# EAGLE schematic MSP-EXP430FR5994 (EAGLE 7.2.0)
DRAWN: Mike Stein; REV: 1.1

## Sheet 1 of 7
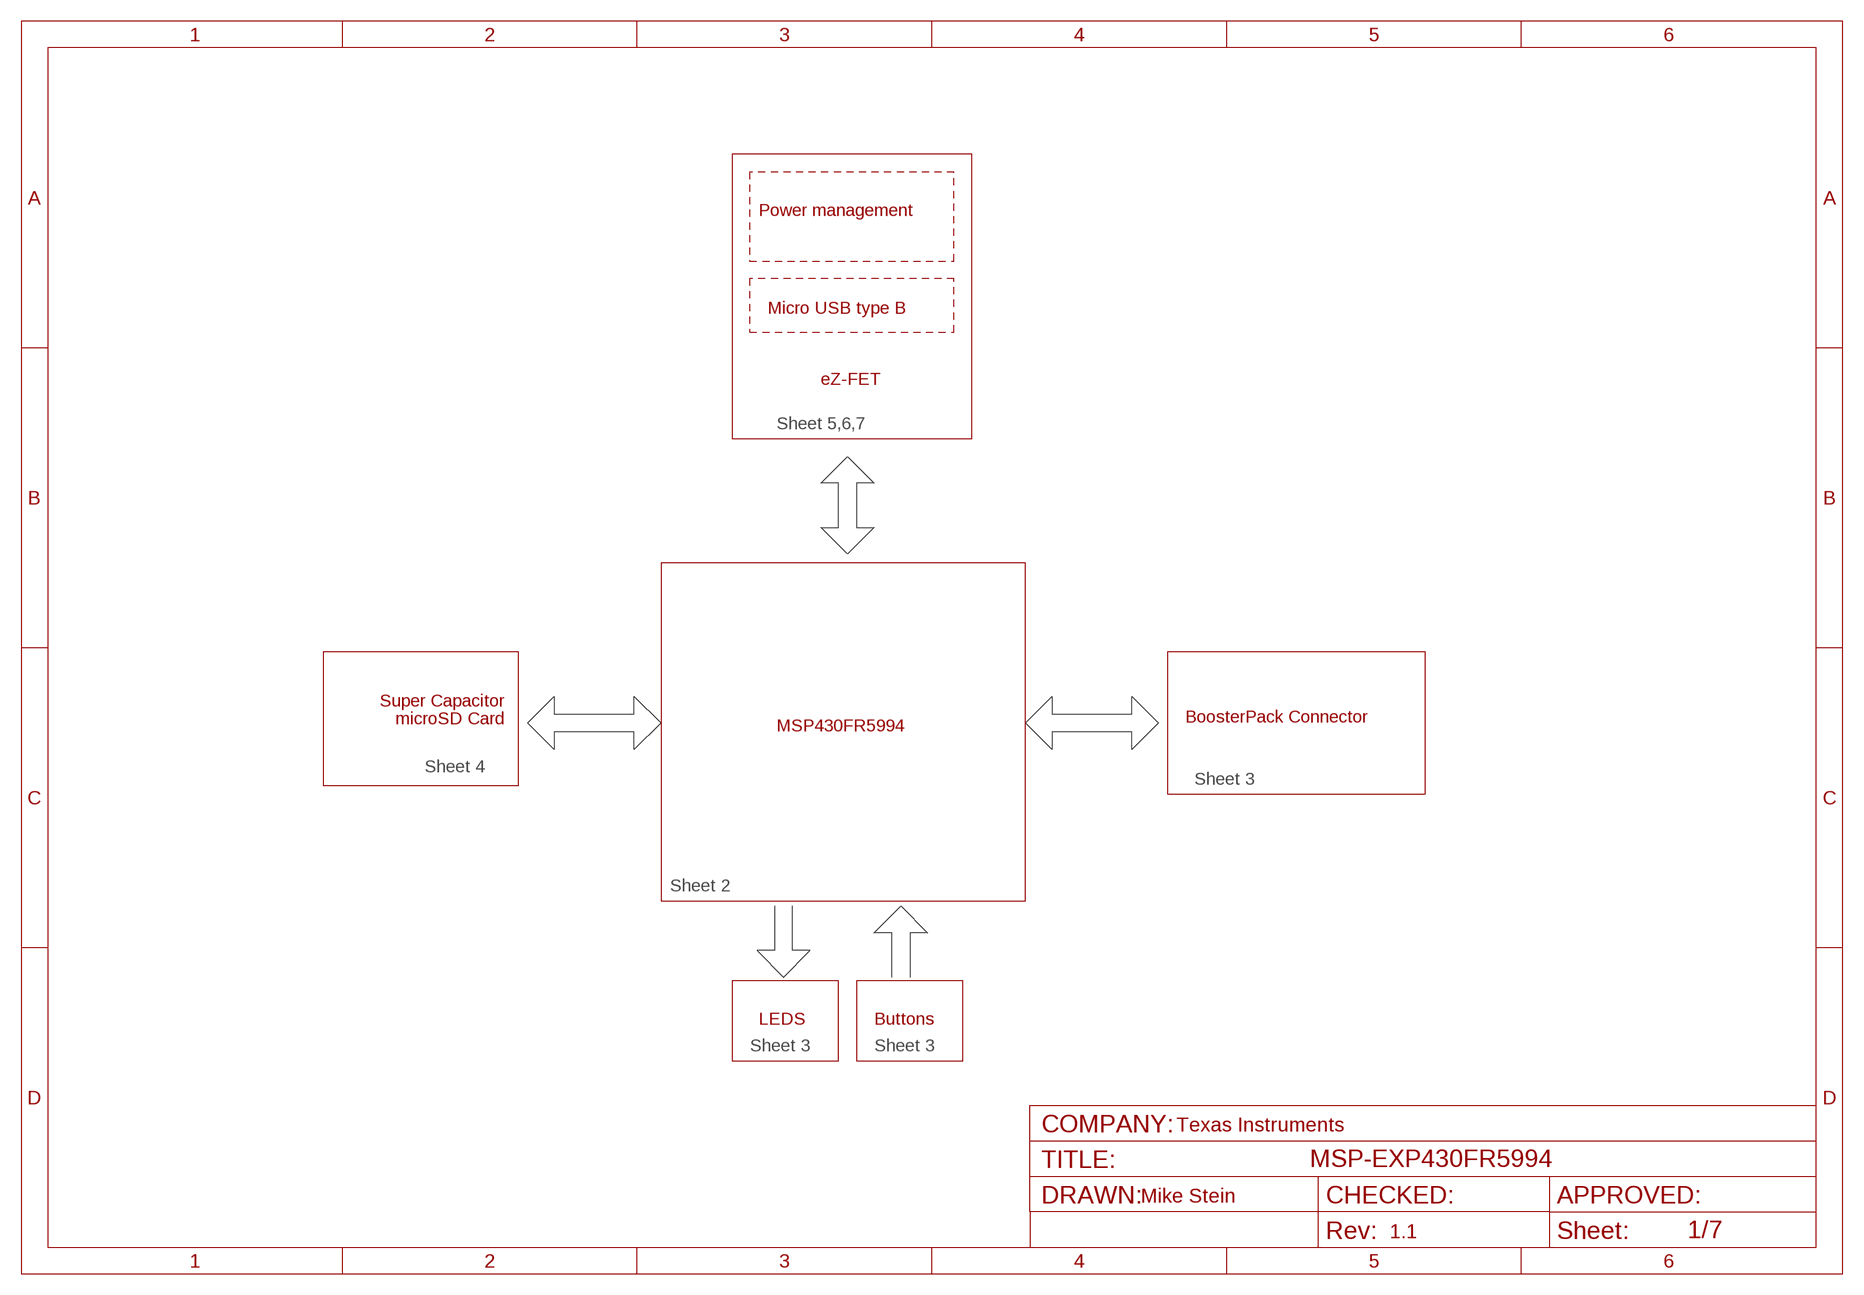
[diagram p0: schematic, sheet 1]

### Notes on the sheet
- Power management
- Micro USB type B
- eZ-FET
- Sheet 5,6,7
- Super Capacitor
- microSD Card
- BoosterPack Connector
- MSP430FR5994
- Sheet 4
- Sheet 3
- Sheet 2
- LEDS | Buttons
- Sheet 3 | Sheet 3
- Texas Instruments

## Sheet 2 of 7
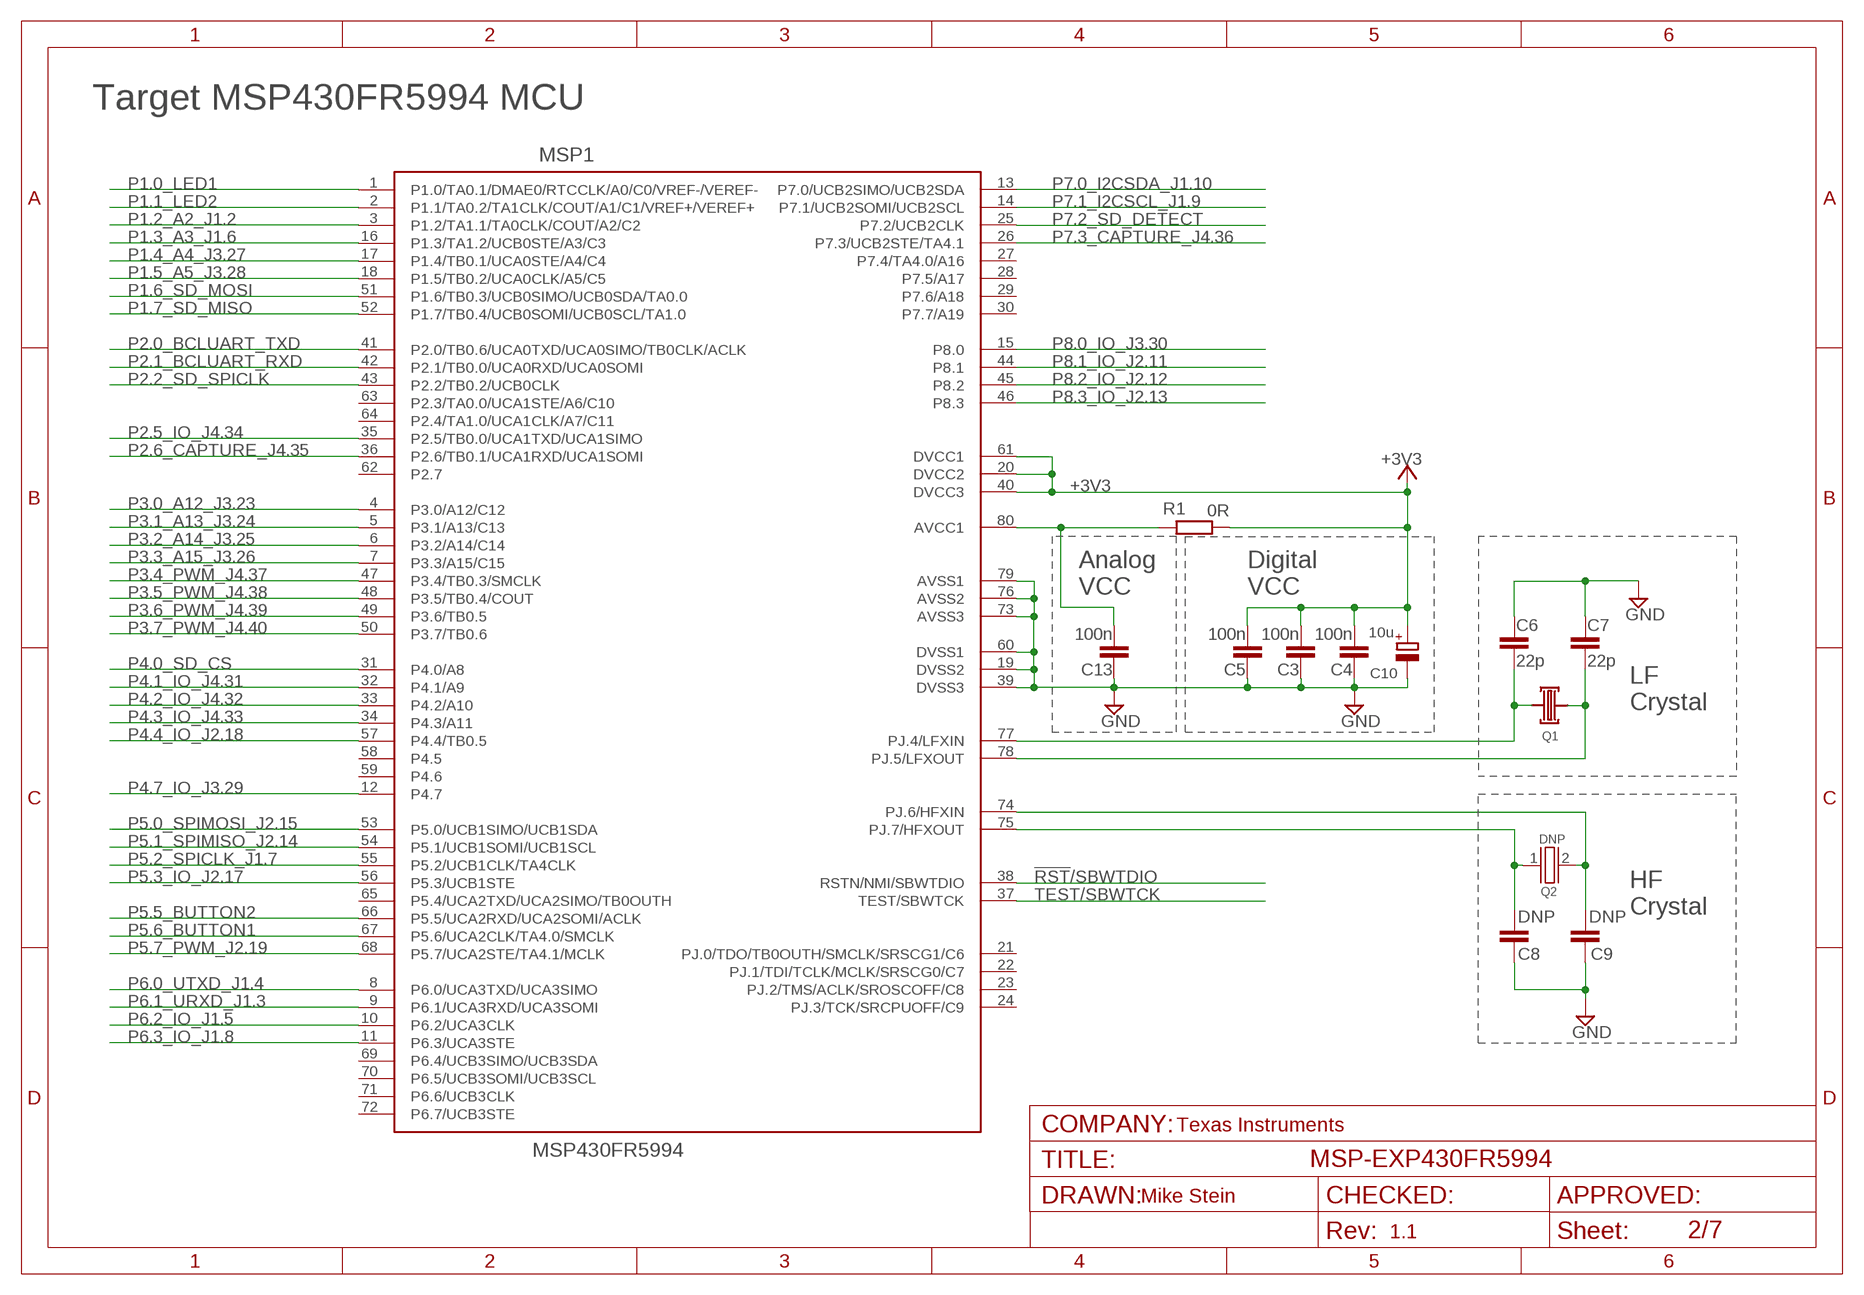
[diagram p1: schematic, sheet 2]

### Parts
C3  100n  C-EUCM0402  [0402]
C4  100n  C-EUCM0402  [0402]
C5  100n  C-EUCM0402  [0402]
C6  22p  C-EUCM0402  [0402]
C7  22p  C-EUCM0402  [0402]
C8  DNP  C-EUCM0402  [0402]
C9  DNP  C-EUCM0402  [0402]
C10  10u  CPOL-EUA/3216-18R  [A/3216-18R]
C13  100n  C-EUCM0402  [0402]
MSP1  MSP430FR5994  [PN80]
Q1  LF_CRYSTAL  [LF_CRYSTAL]
Q2  CRYSTALHF_GENERAL  [HF_XTAL]
R1  0R  R-EU_RM0402  [0402]

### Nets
!RST!/SBWTDIO: MSP1.38(RSTN/NMI/SBWTDIO) ; also sheet 3,6
+3V3: C3.1 C4.1 C5.1 C10.+ MSP1.20(DVCC2) MSP1.40(DVCC3) MSP1.61(DVCC1) R1.1 ; also sheet 3,4,6
N$2: C13.1 MSP1.80(AVCC1) R1.2
N$8: C7.1 MSP1.78(PJ.5/LFXOUT) Q1.2
N$10: C9.1 MSP1.74(PJ.6/HFXIN) Q2.2
N$11: C8.1 MSP1.75(PJ.7/HFXOUT) Q2.1
N$14: C6.1 MSP1.77(PJ.4/LFXIN) Q1.1
P1.0_LED1: MSP1.1(P1.0/TA0.1/DMAE0/RTCCLK/A0/C0/VREF-/VEREF-) ; also sheet 3
P1.1_LED2: MSP1.2(P1.1/TA0.2/TA1CLK/COUT/A1/C1/VREF+/VEREF+) ; also sheet 3
P1.2_A2_J1.2: MSP1.3(P1.2/TA1.1/TA0CLK/COUT/A2/C2) ; also sheet 3
P1.3_A3_J1.6: MSP1.16(P1.3/TA1.2/UCB0STE/A3/C3) ; also sheet 3
P1.4_A4_J3.27: MSP1.17(P1.4/TB0.1/UCA0STE/A4/C4) ; also sheet 3
P1.5_A5_J3.28: MSP1.18(P1.5/TB0.2/UCA0CLK/A5/C5) ; also sheet 3
P1.6_SD_MOSI: MSP1.51(P1.6/TB0.3/UCB0SIMO/UCB0SDA/TA0.0) ; also sheet 4
P1.7_SD_MISO: MSP1.52(P1.7/TB0.4/UCB0SOMI/UCB0SCL/TA1.0) ; also sheet 4
P2.0_BCLUART_TXD: MSP1.41(P2.0/TB0.6/UCA0TXD/UCA0SIMO/TB0CLK/ACLK) ; also sheet 6
P2.1_BCLUART_RXD: MSP1.42(P2.1/TB0.0/UCA0RXD/UCA0SOMI) ; also sheet 6
P2.2_SD_SPICLK: MSP1.43(P2.2/TB0.2/UCB0CLK) ; also sheet 4
P2.5_IO_J4.34: MSP1.35(P2.5/TB0.0/UCA1TXD/UCA1SIMO) ; also sheet 3
P2.6_CAPTURE_J4.35: MSP1.36(P2.6/TB0.1/UCA1RXD/UCA1SOMI) ; also sheet 3
P3.0_A12_J3.23: MSP1.4(P3.0/A12/C12) ; also sheet 3
P3.1_A13_J3.24: MSP1.5(P3.1/A13/C13) ; also sheet 3
P3.2_A14_J3.25: MSP1.6(P3.2/A14/C14) ; also sheet 3
P3.3_A15_J3.26: MSP1.7(P3.3/A15/C15) ; also sheet 3
P3.4_PWM_J4.37: MSP1.47(P3.4/TB0.3/SMCLK) ; also sheet 3
P3.5_PWM_J4.38: MSP1.48(P3.5/TB0.4/COUT) ; also sheet 3
P3.6_PWM_J4.39: MSP1.49(P3.6/TB0.5) ; also sheet 3
P3.7_PWM_J4.40: MSP1.50(P3.7/TB0.6) ; also sheet 3
P4.0_SD_CS: MSP1.31(P4.0/A8) ; also sheet 4
P4.1_IO_J4.31: MSP1.32(P4.1/A9) ; also sheet 3
P4.2_IO_J4.32: MSP1.33(P4.2/A10) ; also sheet 3
P4.3_IO_J4.33: MSP1.34(P4.3/A11) ; also sheet 3
P4.4_IO_J2.18: MSP1.57(P4.4/TB0.5) ; also sheet 3
P4.7_IO_J3.29: MSP1.12(P4.7) ; also sheet 3
P5.0_SPIMOSI_J2.15: MSP1.53(P5.0/UCB1SIMO/UCB1SDA) ; also sheet 3
P5.1_SPIMISO_J2.14: MSP1.54(P5.1/UCB1SOMI/UCB1SCL) ; also sheet 3
P5.2_SPICLK_J1.7: MSP1.55(P5.2/UCB1CLK/TA4CLK) ; also sheet 3
P5.3_IO_J2.17: MSP1.56(P5.3/UCB1STE) ; also sheet 3
P5.5_BUTTON2: MSP1.66(P5.5/UCA2RXD/UCA2SOMI/ACLK) ; also sheet 3
P5.6_BUTTON1: MSP1.67(P5.6/UCA2CLK/TA4.0/SMCLK) ; also sheet 3
P5.7_PWM_J2.19: MSP1.68(P5.7/UCA2STE/TA4.1/MCLK) ; also sheet 3
P6.0_UTXD_J1.4: MSP1.8(P6.0/UCA3TXD/UCA3SIMO) ; also sheet 3
P6.1_URXD_J1.3: MSP1.9(P6.1/UCA3RXD/UCA3SOMI) ; also sheet 3
P6.2_IO_J1.5: MSP1.10(P6.2/UCA3CLK) ; also sheet 3
P6.3_IO_J1.8: MSP1.11(P6.3/UCA3STE) ; also sheet 3
P7.0_I2CSDA_J1.10: MSP1.13(P7.0/UCB2SIMO/UCB2SDA) ; also sheet 3
P7.1_I2CSCL_J1.9: MSP1.14(P7.1/UCB2SOMI/UCB2SCL) ; also sheet 3
P7.2_SD_DETECT: MSP1.25(P7.2/UCB2CLK) ; also sheet 4
P7.3_CAPTURE_J4.36: MSP1.26(P7.3/UCB2STE/TA4.1) ; also sheet 3
P8.0_IO_J3.30: MSP1.15(P8.0) ; also sheet 3
P8.1_IO_J2.11: MSP1.44(P8.1) ; also sheet 3
P8.2_IO_J2.12: MSP1.45(P8.2) ; also sheet 3
P8.3_IO_J2.13: MSP1.46(P8.3) ; also sheet 3
TEST/SBWTCK: MSP1.37(TEST/SBWTCK) ; also sheet 6
TGT_GND: C3.2 C4.2 C5.2 C6.2 C7.2 C8.2 C9.2 C10.- C13.2 MSP1.19(DVSS2) MSP1.39(DVSS3) MSP1.60(DVSS1) MSP1.73(AVSS3) MSP1.76(AVSS2) MSP1.79(AVSS1) ; supply symbol labelled GND ; also sheet 3,4,6

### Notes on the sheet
- Target MSP430FR5994 MCU
- Analog | Digital
- VCC | VCC
- LF
- Crystal
- DNP
- HF
- Crystal
- Texas Instruments

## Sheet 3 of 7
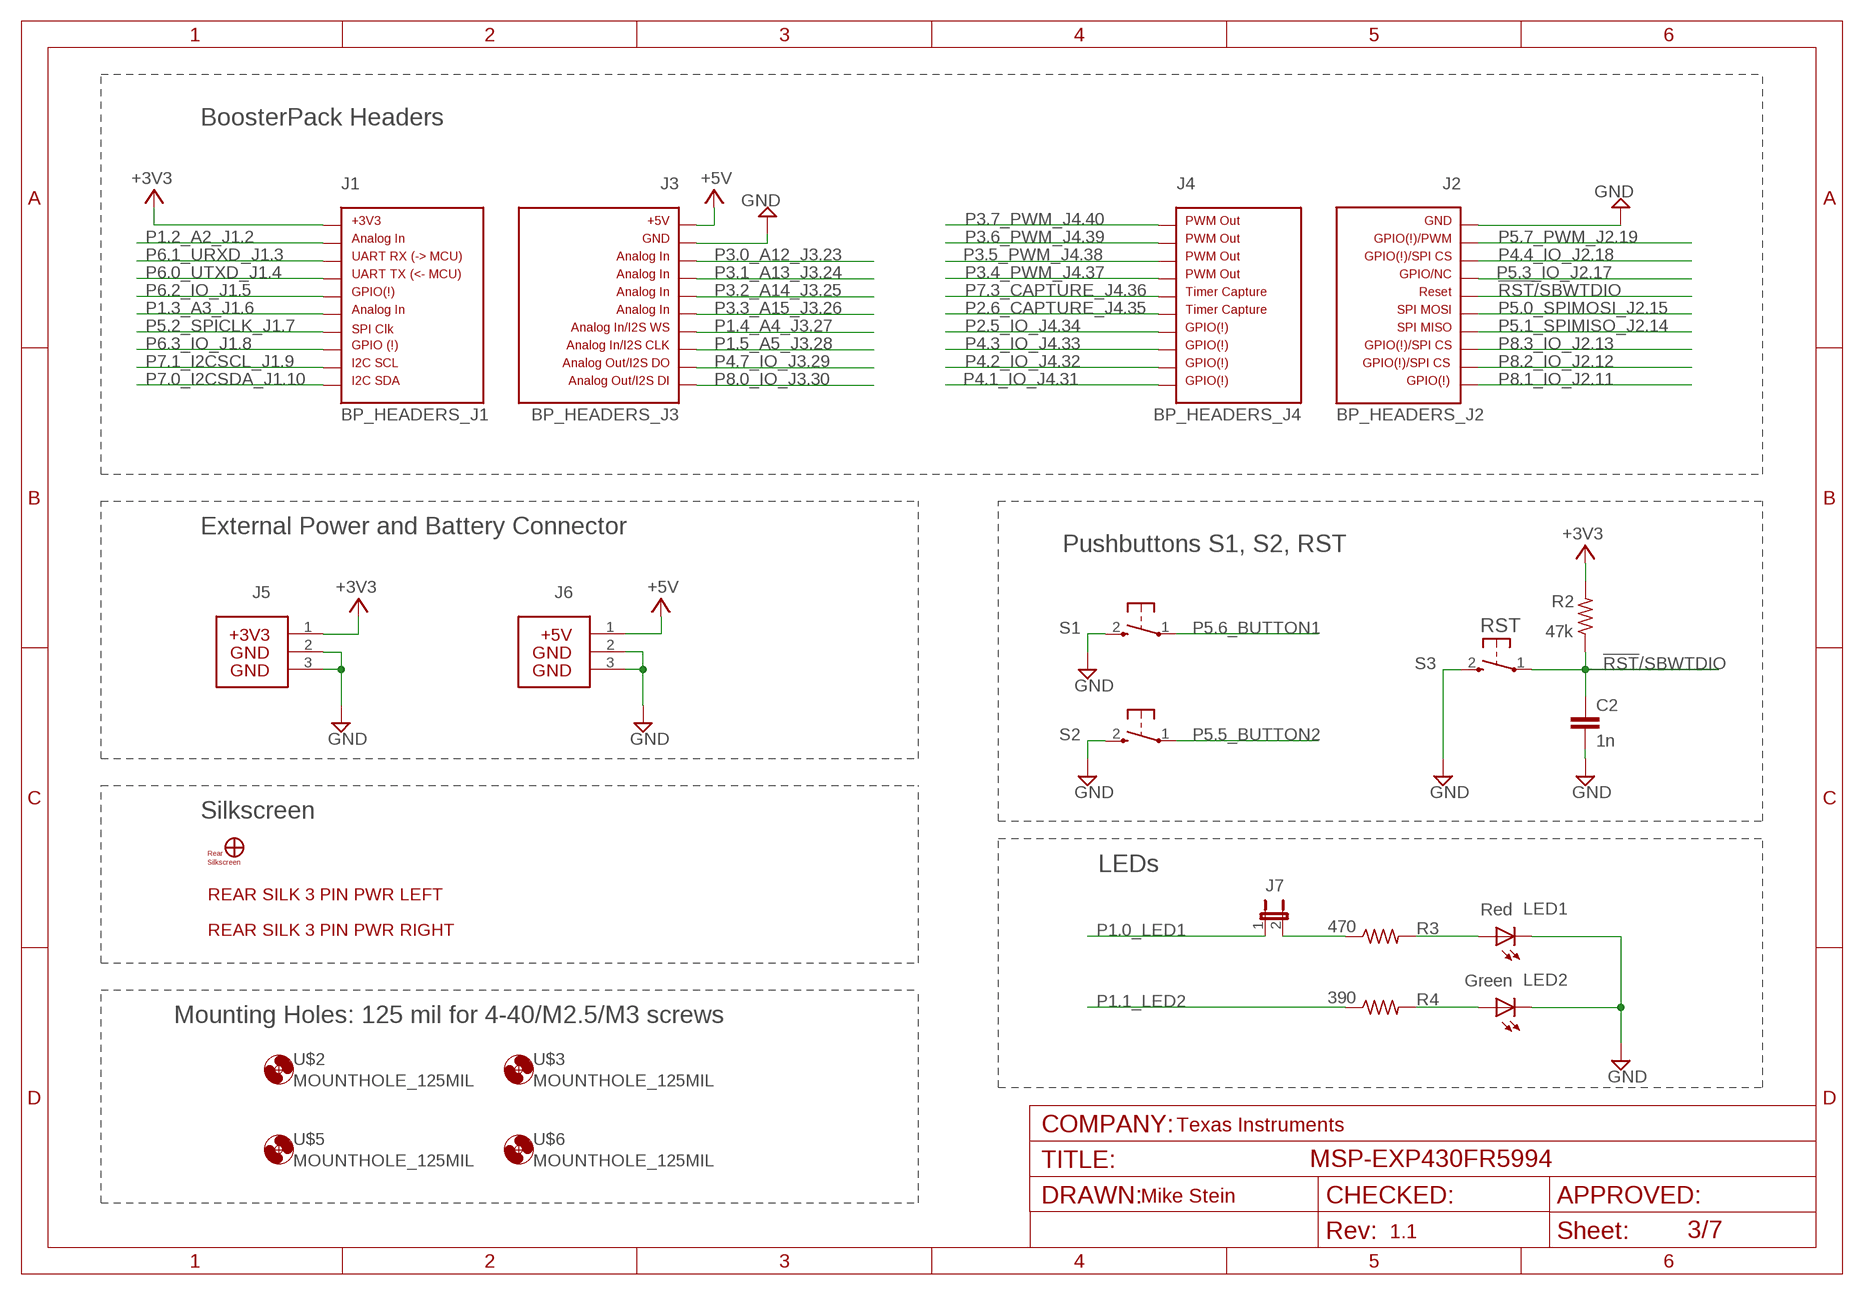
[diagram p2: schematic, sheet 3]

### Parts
C2  1n  C-EUCM0402  [0402]
J1  BP_HEADERS_J1  [J1]
J2  BP_HEADERS_J2  [J2]
J3  BP_HEADERS_J3  [J3]
J4  BP_HEADERS_J4  [J4]
J5  HEADER 1X03  BP_HEADERS_PWR_3V3100-TH  [3PIN_PWR_3V3]
J6  BP_HEADERS_PWR_5V  [3PIN_PWR_5V]
J7  JUMPER1X02  [1X02]
LED1  Red  CHIP-LED  [LED0805]
LED2  Green  CHIP-LED  [LED0805]
R2  47k  R-US_RM0402  [0402]
R3  470  R-US_RM0402  [0402]
R4  390  R-US_RM0402  [0402]
S1  PB  [PBTH]
S2  PB  [PBTH]
S3  PB  [PBTH]
U$1  FR5994_REARSILK_REV1_0  [FR5994_REARSILK_REV1_0]
U$2  MOUNTHOLE_125MIL  [MOUNTHOLE_125MIL]
U$3  MOUNTHOLE_125MIL  [MOUNTHOLE_125MIL]
U$5  MOUNTHOLE_125MIL  [MOUNTHOLE_125MIL]
U$6  MOUNTHOLE_125MIL  [MOUNTHOLE_125MIL]
U$7  MIKE_TM  [MIKE_TM]
U$8  BP_3PIN_SILK  [3PIN_PWR_SILK]
U$10  BP_3PIN_SILK_RT  [3PIN_PWR_SILK_RT]

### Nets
!RST!/SBWTDIO: C2.1 J2.16 R2.1 S3.1(P) ; also sheet 2,6
+3V3: J1.1 J5.1 R2.2 ; also sheet 2,4,6
+5V: J3.21 J6.1 ; also sheet 6
N$4: LED2.A R4.2
N$6: J7.2 R3.1
N$7: LED1.A R3.2
P1.0_LED1: J7.1 ; also sheet 2
P1.1_LED2: R4.1 ; also sheet 2
P1.2_A2_J1.2: J1.2 ; also sheet 2
P1.3_A3_J1.6: J1.6 ; also sheet 2
P1.4_A4_J3.27: J3.27 ; also sheet 2
P1.5_A5_J3.28: J3.28 ; also sheet 2
P2.5_IO_J4.34: J4.34 ; also sheet 2
P2.6_CAPTURE_J4.35: J4.35 ; also sheet 2
P3.0_A12_J3.23: J3.23 ; also sheet 2
P3.1_A13_J3.24: J3.24 ; also sheet 2
P3.2_A14_J3.25: J3.25 ; also sheet 2
P3.3_A15_J3.26: J3.26 ; also sheet 2
P3.4_PWM_J4.37: J4.37 ; also sheet 2
P3.5_PWM_J4.38: J4.38 ; also sheet 2
P3.6_PWM_J4.39: J4.39 ; also sheet 2
P3.7_PWM_J4.40: J4.40 ; also sheet 2
P4.1_IO_J4.31: J4.31 ; also sheet 2
P4.2_IO_J4.32: J4.32 ; also sheet 2
P4.3_IO_J4.33: J4.33 ; also sheet 2
P4.4_IO_J2.18: J2.18 ; also sheet 2
P4.7_IO_J3.29: J3.29 ; also sheet 2
P5.0_SPIMOSI_J2.15: J2.15 ; also sheet 2
P5.1_SPIMISO_J2.14: J2.14 ; also sheet 2
P5.2_SPICLK_J1.7: J1.7 ; also sheet 2
P5.3_IO_J2.17: J2.17 ; also sheet 2
P5.5_BUTTON2: S2.1(P) ; also sheet 2
P5.6_BUTTON1: S1.1(P) ; also sheet 2
P5.7_PWM_J2.19: J2.19 ; also sheet 2
P6.0_UTXD_J1.4: J1.4 ; also sheet 2
P6.1_URXD_J1.3: J1.3 ; also sheet 2
P6.2_IO_J1.5: J1.5 ; also sheet 2
P6.3_IO_J1.8: J1.8 ; also sheet 2
P7.0_I2CSDA_J1.10: J1.10 ; also sheet 2
P7.1_I2CSCL_J1.9: J1.9 ; also sheet 2
P7.3_CAPTURE_J4.36: J4.36 ; also sheet 2
P8.0_IO_J3.30: J3.30 ; also sheet 2
P8.1_IO_J2.11: J2.11 ; also sheet 2
P8.2_IO_J2.12: J2.12 ; also sheet 2
P8.3_IO_J2.13: J2.13 ; also sheet 2
TGT_GND: C2.2 J2.20 J3.22 J5.2 J5.3 J6.2 J6.3 LED1.C LED2.C S1.2(S) S2.2(S) S3.2(S) ; supply symbol labelled GND ; also sheet 2,4,6

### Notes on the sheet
- BoosterPack Headers
- External Power and Battery Connector
- Pushbuttons S1, S2, RST
- RST
- Silkscreen
- LEDs
- Mounting Holes: 125 mil for 4-40/M2.5/M3 screws
- Texas Instruments

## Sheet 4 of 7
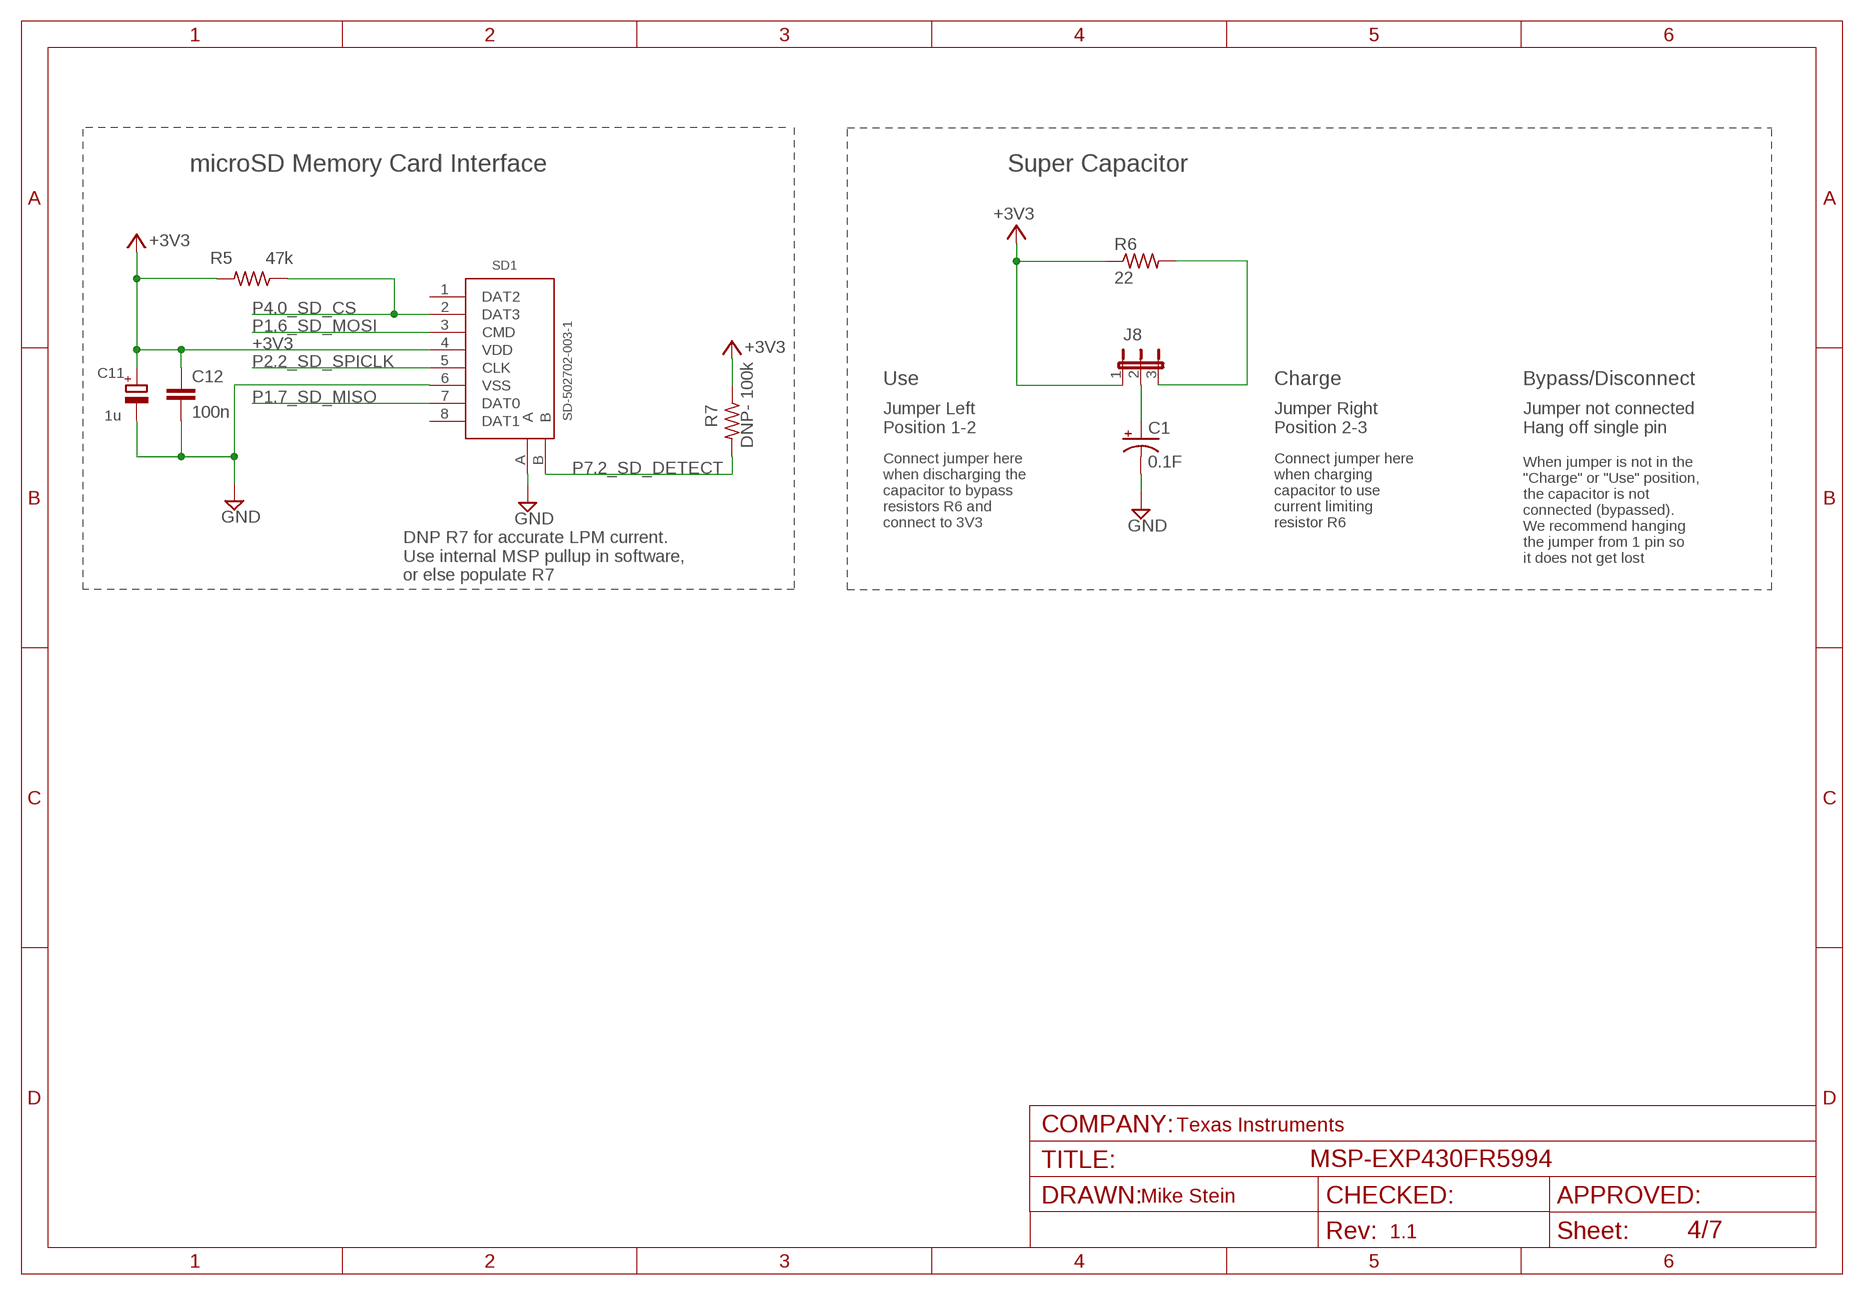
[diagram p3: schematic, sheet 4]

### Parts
C1  0.1F  PANASONIC_SUPERCAP  [PANASONIC_SUPERCAP]
C11  1u  CPOL-EUA/3216-18R  [A/3216-18R]
C12  100n  C-EUCM0402  [0402]
J8  JUMPER1X03  [1X03]
R5  47k  R-US_RM0402  [0402]
R6  22  R-US_R3216  [R3216]
R7  DNP- 100k  R-US_RM0402  [0402]
SD1  SD-502702-003-1  [SD-502702-003]

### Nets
+3V3: C11.+ C12.1 J8.1 R5.2 R6.1 R7.1 SD1.4(VDD) ; also sheet 2,3,6
N$3: C1.+ J8.2
N$17: J8.3 R6.2
P1.6_SD_MOSI: SD1.3(CMD) ; also sheet 2
P1.7_SD_MISO: SD1.7(DAT0) ; also sheet 2
P2.2_SD_SPICLK: SD1.5(CLK) ; also sheet 2
P4.0_SD_CS: R5.1 SD1.2(DAT3) ; also sheet 2
P7.2_SD_DETECT: R7.2 SD1.B ; also sheet 2
TGT_GND: C1.- C11.- C12.2 SD1.6(VSS) SD1.A ; supply symbol labelled GND ; also sheet 2,3,6
Unconnected: SD1.1(DAT2) SD1.8(DAT1)

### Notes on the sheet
- microSD Memory Card Interface | Super Capacitor
- Use | Charge | Bypass/Disconnect
- Jumper Left
  Position 1-2
- Jumper Right
  Position 2-3
- Jumper not connected
  Hang off single pin
- Connect jumper here
  when discharging the
  capacitor to bypass
  resistors R6 and
  connect to 3V3
- Connect jumper here
  when charging
  capacitor to use
  current limiting
  resistor R6
- When jumper is not in the
  "Charge" or "Use" position,
  the capacitor is not
  connected (bypassed).
  We recommend hanging
  the jumper from 1 pin so
  it does not get lost
- DNP R7 for accurate LPM current. 
  Use internal MSP pullup in software, 
  or else populate R7
- Texas Instruments

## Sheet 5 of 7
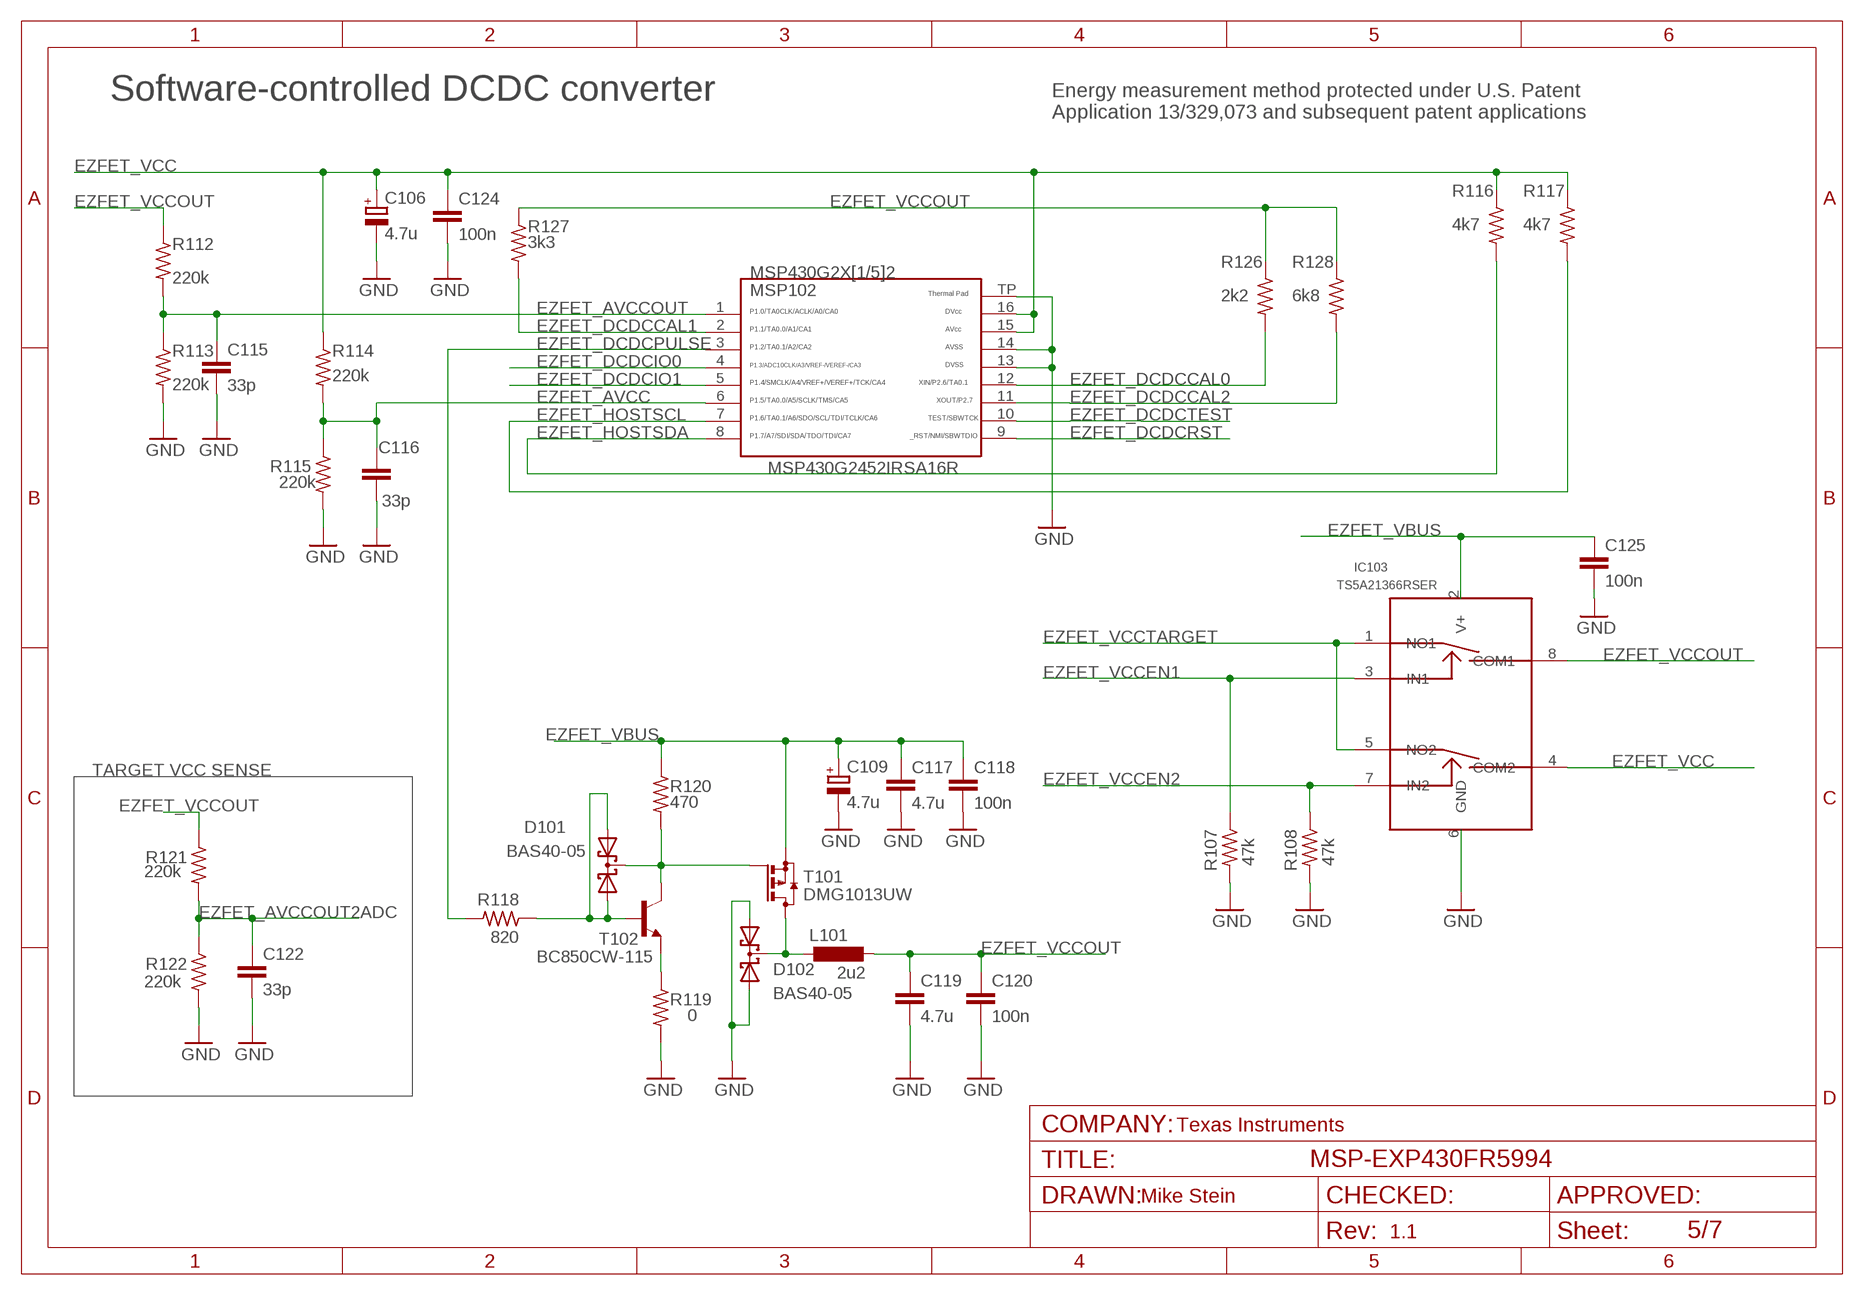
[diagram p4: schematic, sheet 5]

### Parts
C106  4.7u  CPOL-EUA/3216-18R  [A/3216-18R]
C109  4.7u  CPOL-EUA/3216-18R  [A/3216-18R]
C115  33p  C-EUCM0402  [0402]
C116  33p  C-EUCM0402  [0402]
C117  4.7u  C-EUC0603  [C0603]
C118  100n  C-EUCM0402  [0402]
C119  4.7u  C-EUC0603  [C0603]
C120  100n  C-EUCM0402  [0402]
C122  33p  C-EUCM0402  [0402]
C124  100n  C-EUCM0402  [0402]
C125  100n  C-EUCM0402  [0402]
D101  BAS40-05  BAS40-05W  [SOT323]
D102  BAS40-05  BAS40-05W  [SOT323]
IC103  TS5A21366RSER  [UQFN_RSE]
L101  2u2  L-EUL3216C  [L3216C]
MSP102  MSP430G2452IRSA16R  G2X[1/5]2---RSA16  [RSA16]
R107  47k  R-US_RM0402  [0402]
R108  47k  R-US_RM0402  [0402]
R112  220k  R-US_RM0402  [0402]
R113  220k  R-US_RM0402  [0402]
R114  220k  R-US_RM0402  [0402]
R115  220k  R-US_RM0402  [0402]
R116  4k7  R-US_RM0402  [0402]
R117  4k7  R-US_RM0402  [0402]
R118  820  R-US_RM0402  [0402]
R119  0  R-US_RM0402  [0402]
R120  470  R-US_RM0402  [0402]
R121  220k  R-US_RM0402  [0402]
R122  220k  R-US_RM0402  [0402]
R126  2k2  R-US_RM0402  [0402]
R127  3k3  R-US_RM0402  [0402]
R128  6k8  R-US_RM0402  [0402]
T101  DMG1013UW  [SOT323]
T102  BC850CW-115  [SOT323]

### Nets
EZFET_AVCC: C116.2 MSP102.6 R114.2 R115.1
EZFET_AVCCOUT: C115.2 MSP102.1 R112.2 R113.1
EZFET_AVCCOUT2ADC: C122.2 R121.2 R122.1 ; also sheet 6
EZFET_DCDCCAL0: MSP102.12 R126.2
EZFET_DCDCCAL1: MSP102.2 R127.2
EZFET_DCDCCAL2: MSP102.11 R128.2
EZFET_DCDCIO0: MSP102.4 ; also sheet 6
EZFET_DCDCIO1: MSP102.5 ; also sheet 6
EZFET_DCDCPULSE: MSP102.3 R118.2 ; also sheet 6
EZFET_DCDCRST: MSP102.9 ; also sheet 6,7
EZFET_DCDCTEST: MSP102.10 ; also sheet 6,7
EZFET_HOSTSCL: MSP102.7 R117.2 ; also sheet 6
EZFET_HOSTSDA: MSP102.8 R116.2 ; also sheet 6
EZFET_VBUS: C109.+ C117.1 C118.1 C125.1 IC103.2(V+) R120.1 T101.2(S) ; also sheet 6,7
EZFET_VCC: C106.+ C124.1 IC103.4(COM2) MSP102.15 MSP102.16 R114.1 R116.1 R117.1 ; also sheet 6,7
EZFET_VCCEN1: IC103.3(IN1) R107.1 ; also sheet 6
EZFET_VCCEN2: IC103.7(IN2) R108.1 ; also sheet 6
EZFET_VCCOUT: C119.1 C120.1 IC103.8(COM1) L101.2 R112.1 R121.1 R126.1 R127.1 R128.1
EZFET_VCCTARGET: IC103.1(NO1) IC103.5(NO2) ; also sheet 6
GND: C106.- C109.- C115.1 C116.1 C117.2 C118.2 C119.2 C120.2 C122.1 C124.2 C125.2 D102.1(A1) D102.2(A2) IC103.6(GND) MSP102.13 MSP102.14 MSP102.TP R107.2 R108.2 R113.2 R115.2 R119.2 R122.2 ; also sheet 6,7
N$12: R119.1 T102.2(E)
N$13: D101.1(A1) D101.2(A2) R118.1 T102.1(B)
N$15: D102.3(C) L101.1 T101.3(D)
N$16: D101.3(C) R120.2 T101.1(G) T102.3(C)

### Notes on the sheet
- Software-controlled DCDC converter
- Energy measurement method protected under U.S. Patent 
  Application 13/329,073 and subsequent patent applications
- MSP430G2452IRSA16R
- TARGET VCC SENSE
- Texas Instruments

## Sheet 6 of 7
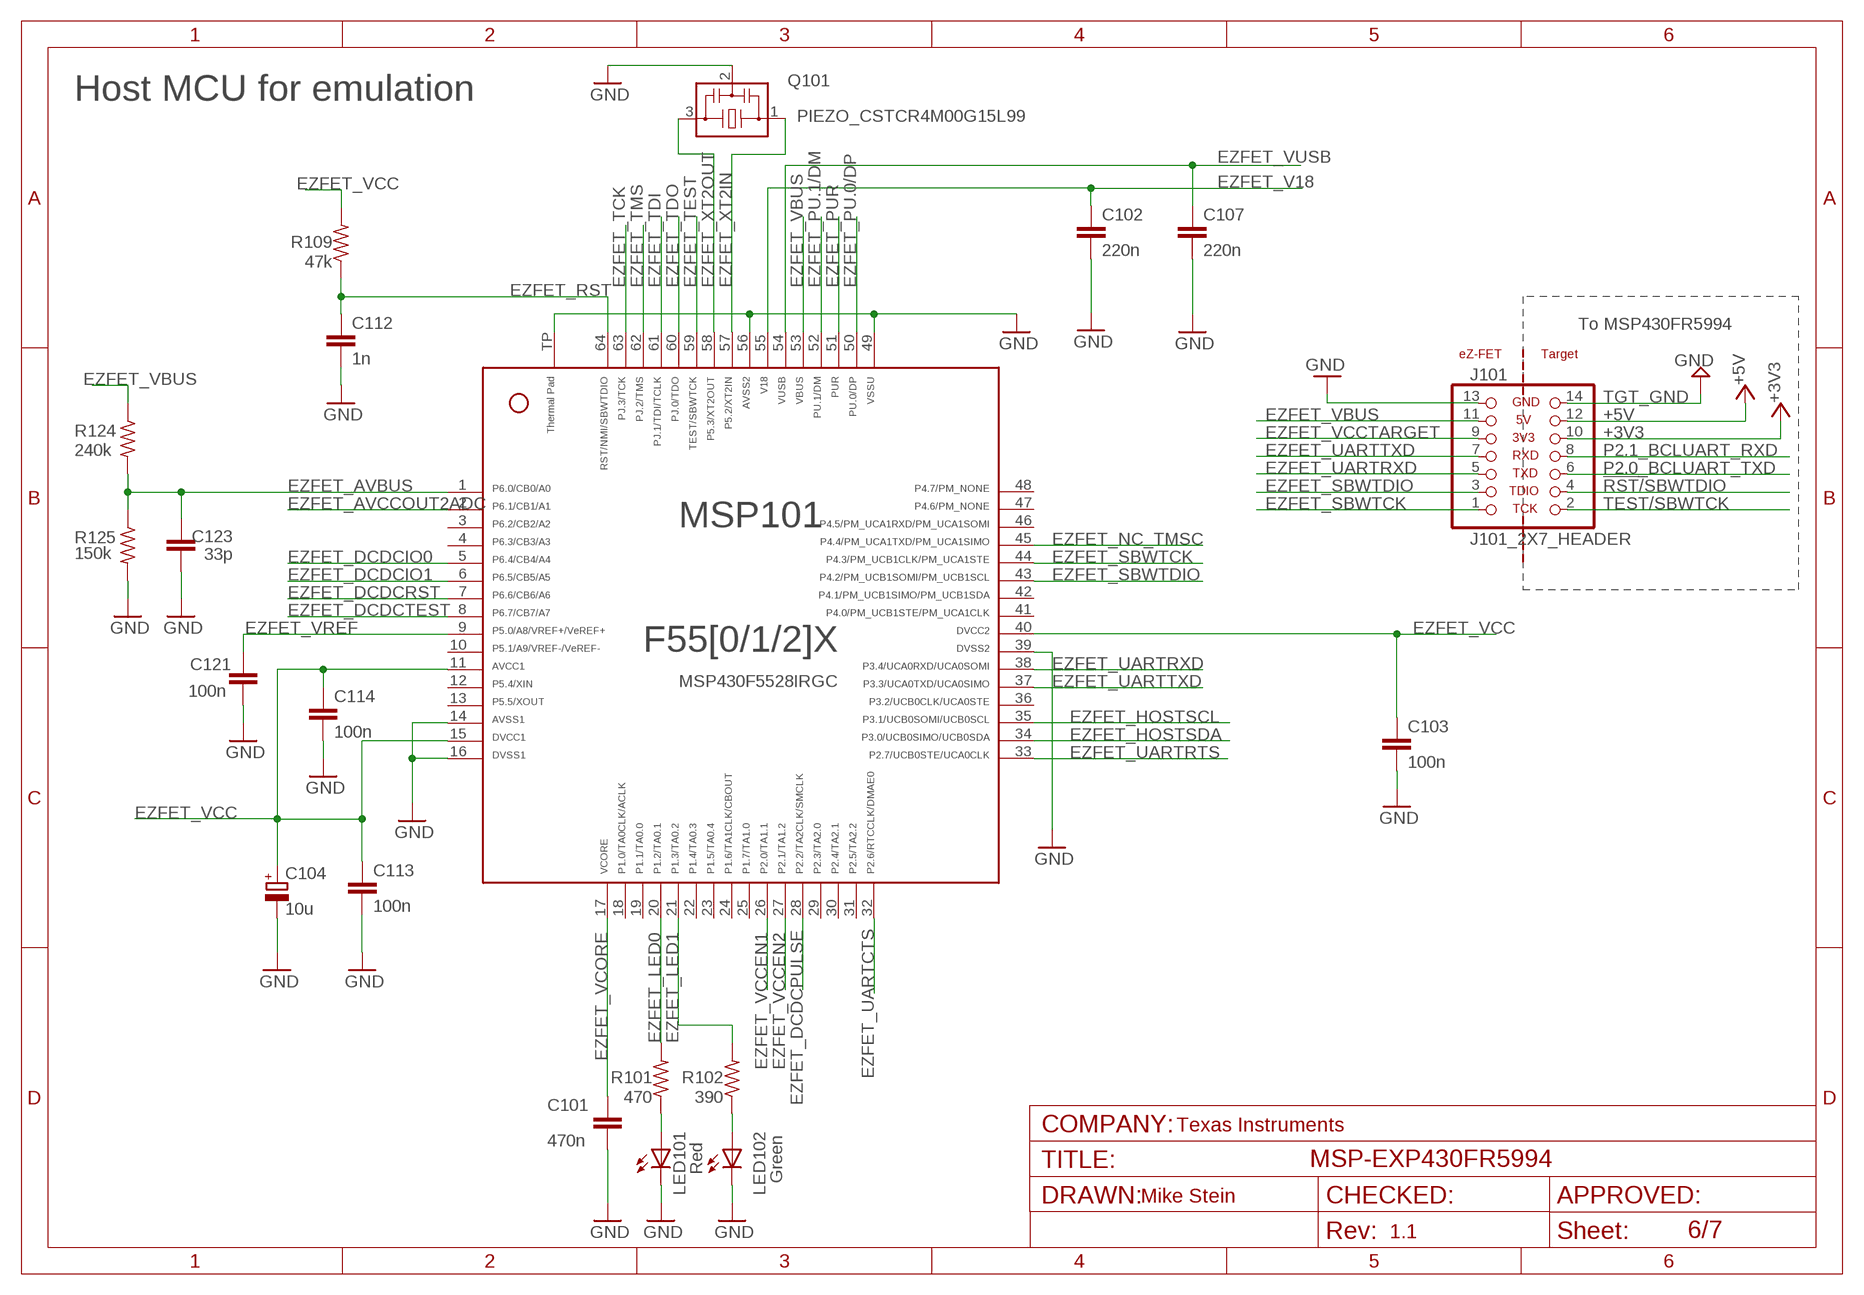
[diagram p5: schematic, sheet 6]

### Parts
C101  470n  C-EUCM0402  [0402]
C102  220n  C-EUCM0402  [0402]
C103  100n  C-EUCM0402  [0402]
C104  10u  CPOL-EUA/3216-18R  [A/3216-18R]
C107  220n  C-EUCM0402  [0402]
C112  1n  C-EUCM0402  [0402]
C113  100n  C-EUCM0402  [0402]
C114  100n  C-EUCM0402  [0402]
C121  100n  C-EUCM0402  [0402]
C123  33p  C-EUCM0402  [0402]
J101  J101_2X7_HEADER  [J101]
LED101  Red  CHIP-LED  [LED0805]
LED102  Green  CHIP-LED  [LED0805]
MSP101  MSP430F5528IRGC  F55[0/1/2]X---RGC64  [RGC64]
Q101  PIEZO_CSTCR4M00G15L99  CSTCR4M  [CSTCR4M]
R101  470  R-US_RM0402  [0402]
R102  390  R-US_RM0402  [0402]
R109  47k  R-US_RM0402  [0402]
R124  240k  R-US_RM0402  [0402]
R125  150k  R-US_RM0402  [0402]

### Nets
!RST!/SBWTDIO: J101.4 ; also sheet 2,3
+3V3: J101.10 ; also sheet 2,3,4
+5V: J101.12 ; also sheet 3
EZFET_AVBUS: C123.2 MSP101.1 R124.2 R125.1
EZFET_AVCCOUT2ADC: MSP101.2 ; also sheet 5
EZFET_DCDCIO0: MSP101.5 ; also sheet 5
EZFET_DCDCIO1: MSP101.6 ; also sheet 5
EZFET_DCDCPULSE: MSP101.28 ; also sheet 5
EZFET_DCDCRST: MSP101.7 ; also sheet 5,7
EZFET_DCDCTEST: MSP101.8 ; also sheet 5,7
EZFET_HOSTSCL: MSP101.35 ; also sheet 5
EZFET_HOSTSDA: MSP101.34 ; also sheet 5
EZFET_LED0: MSP101.20 R101.2
EZFET_LED1: MSP101.21 R102.2
EZFET_NC_TMSC: MSP101.45
EZFET_PU.0/DP: MSP101.50 ; also sheet 7
EZFET_PU.1/DM: MSP101.52 ; also sheet 7
EZFET_PUR: MSP101.51 ; also sheet 7
EZFET_RST: C112.1 MSP101.64 R109.1 ; also sheet 7
EZFET_SBWTCK: J101.1 MSP101.44
EZFET_SBWTDIO: J101.3 MSP101.43
EZFET_TCK: MSP101.63 ; also sheet 7
EZFET_TDI: MSP101.61 ; also sheet 7
EZFET_TDO: MSP101.60 ; also sheet 7
EZFET_TEST: MSP101.59 ; also sheet 7
EZFET_TMS: MSP101.62 ; also sheet 7
EZFET_UARTCTS: MSP101.32
EZFET_UARTRTS: MSP101.33
EZFET_UARTRXD: J101.5 MSP101.38
EZFET_UARTTXD: J101.7 MSP101.37
EZFET_V18: C102.1 MSP101.55
EZFET_VBUS: J101.11 MSP101.53 R124.1 ; also sheet 5,7
EZFET_VCC: C103.1 C104.+ C113.1 C114.1 MSP101.11 MSP101.15 MSP101.40 R109.2 ; also sheet 5,7
EZFET_VCCEN1: MSP101.26 ; also sheet 5
EZFET_VCCEN2: MSP101.27 ; also sheet 5
EZFET_VCCTARGET: J101.9 ; also sheet 5
EZFET_VCORE: C101.1 MSP101.17
EZFET_VREF: C121.1 MSP101.9
EZFET_VUSB: C107.1 MSP101.54
EZFET_XT2IN: MSP101.57 Q101.1
EZFET_XT2OUT: MSP101.58 Q101.3
GND: C101.2 C102.2 C103.2 C104.- C107.2 C112.2 C113.2 C114.2 C121.2 C123.1 J101.13 LED101.C LED102.C MSP101.14 MSP101.16 MSP101.39 MSP101.49 MSP101.56 MSP101.TP Q101.2 R125.2 ; also sheet 5,7
N$9: LED101.A R101.1
N$20: LED102.A R102.1
P2.0_BCLUART_TXD: J101.6 ; also sheet 2
P2.1_BCLUART_RXD: J101.8 ; also sheet 2
TEST/SBWTCK: J101.2 ; also sheet 2
TGT_GND: J101.14 ; supply symbol labelled GND ; also sheet 2,3,4
Unconnected: MSP101.3 MSP101.4 MSP101.10 MSP101.12 MSP101.13 MSP101.18 MSP101.19 MSP101.22 MSP101.23 MSP101.24 MSP101.25 MSP101.29 MSP101.30 MSP101.31 MSP101.36 MSP101.41 MSP101.42 MSP101.46 MSP101.47 MSP101.48

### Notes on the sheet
- Host MCU for emulation
- To MSP430FR5994
- MSP430F5528IRGC
- Texas Instruments

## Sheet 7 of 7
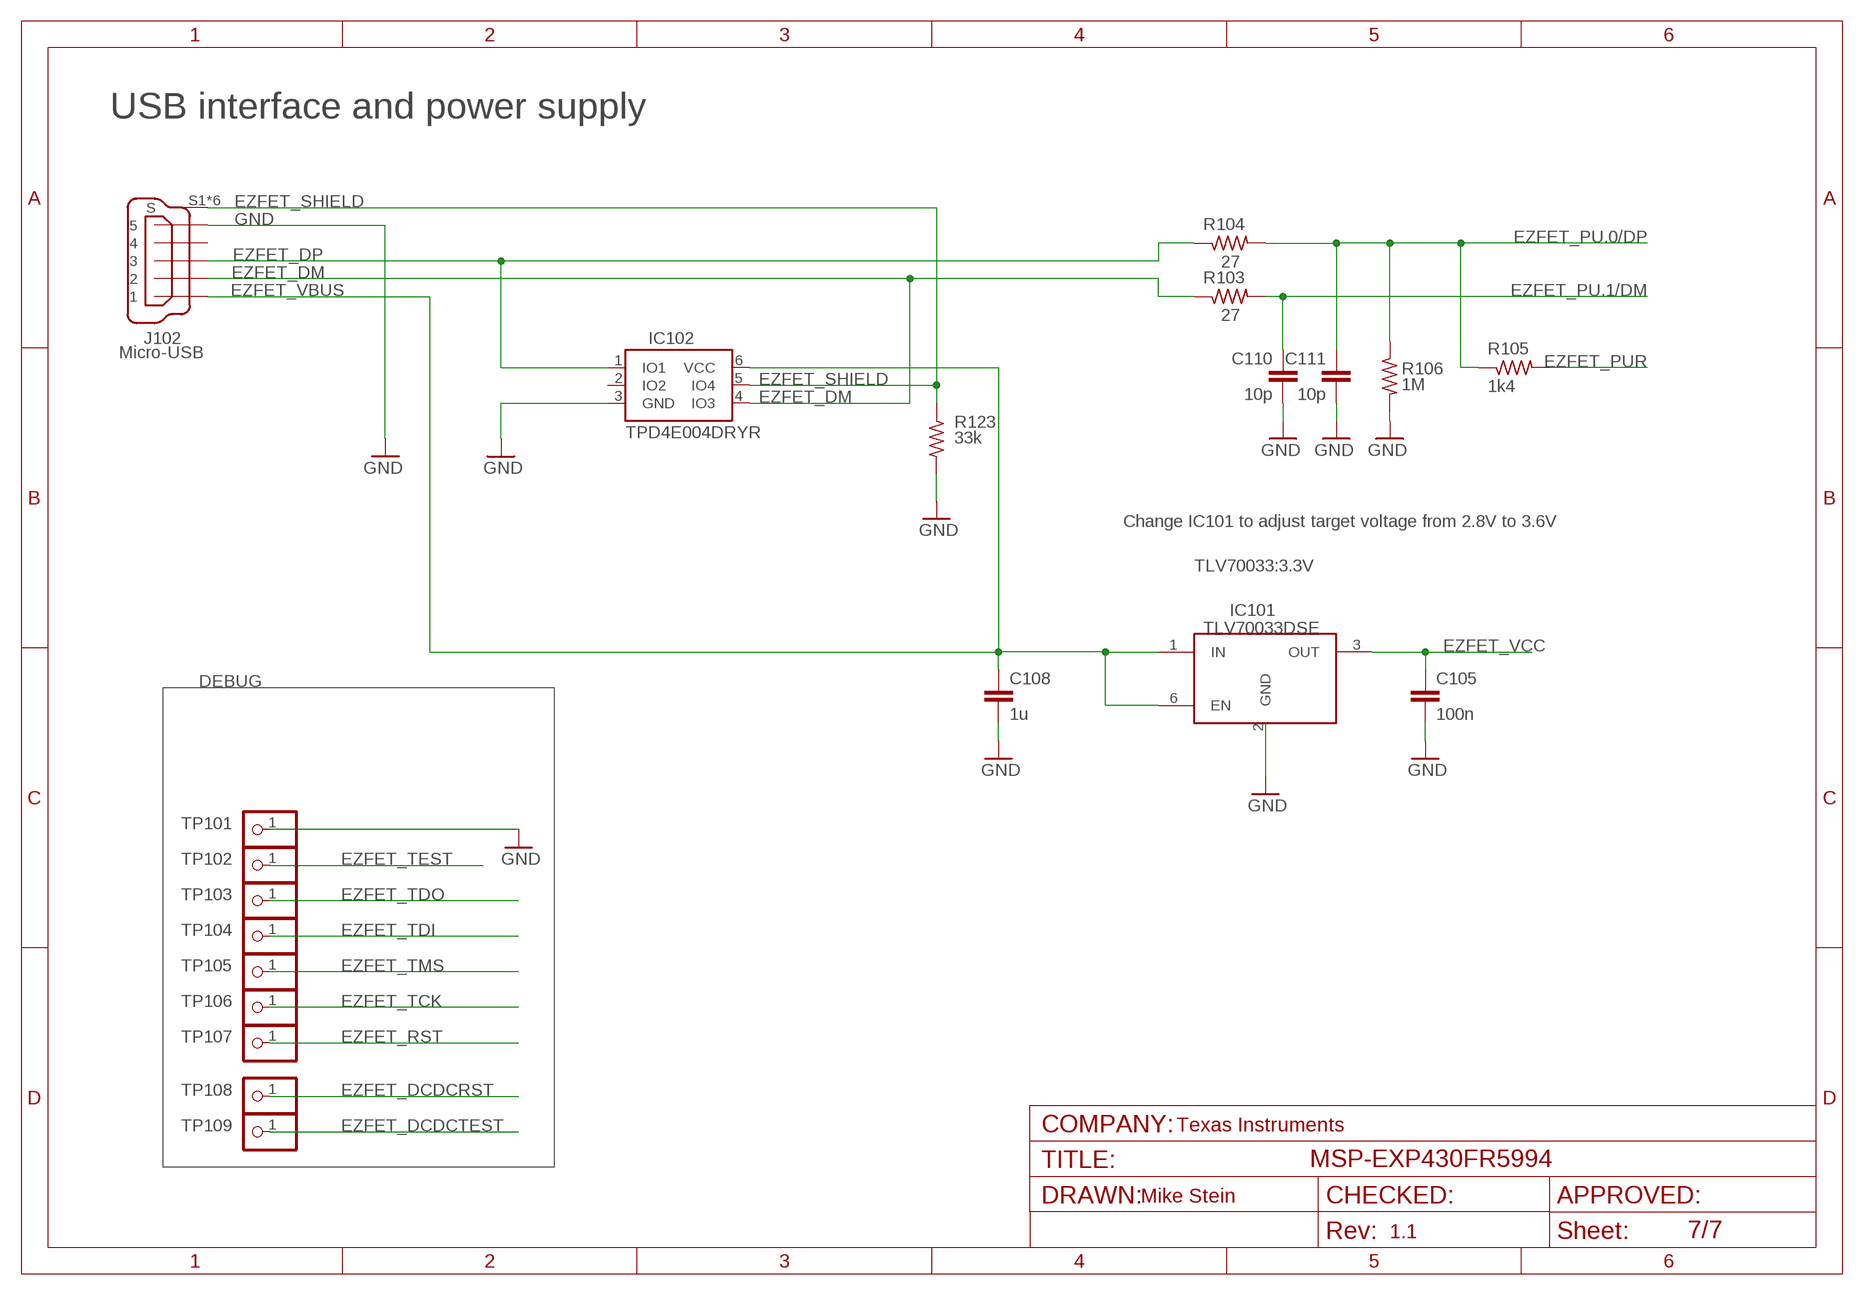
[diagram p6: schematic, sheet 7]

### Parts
C105  100n  C-EUCM0402  [0402]
C108  1u  C-EUC0603  [C0603]
C110  10p  C-EUCM0402  [0402]
C111  10p  C-EUCM0402  [0402]
IC101  TLV70033DSE  [WSON_DSE]
IC102  TPD4E004DRYR  TPD4E004  [SON(DRY)6]
J102  Micro-USB  EZFET_MINI-USB-  [EZFET_UX62M-B-5P]
R103  27  R-US_RM0402  [0402]
R104  27  R-US_RM0402  [0402]
R105  1k4  R-US_RM0402  [0402]
R106  1M  R-US_RM0402  [0402]
R123  33k  R-US_RM0402  [0402]
TP101  TEST_PIN2  PINHD-1X1  [1X01]
TP102  TEST_PIN2  PINHD-1X1  [1X01]
TP103  TEST_PIN2  PINHD-1X1  [1X01]
TP104  TEST_PIN2  PINHD-1X1  [1X01]
TP105  TEST_PIN2  PINHD-1X1  [1X01]
TP106  TEST_PIN2  PINHD-1X1  [1X01]
TP107  TEST_PIN2  PINHD-1X1  [1X01]
TP108  TEST_PIN2  PINHD-1X1  [1X01]
TP109  TEST_PIN2  PINHD-1X1  [1X01]

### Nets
EZFET_DCDCRST: TP108.1 ; also sheet 5,6
EZFET_DCDCTEST: TP109.1 ; also sheet 5,6
EZFET_DM: IC102.4(IO3) J102.2 R103.1
EZFET_DP: IC102.1(IO1) J102.3 R104.1
EZFET_PU.0/DP: C111.1 R104.2 R105.1 R106.1 ; also sheet 6
EZFET_PU.1/DM: C110.1 R103.2 ; also sheet 6
EZFET_PUR: R105.2 ; also sheet 6
EZFET_RST: TP107.1 ; also sheet 6
EZFET_SHIELD: IC102.5(IO4) J102.S1(S) J102.S2(S) J102.S3(S) J102.S4(S) J102.S5(S) J102.S6(S) R123.1
EZFET_TCK: TP106.1 ; also sheet 6
EZFET_TDI: TP104.1 ; also sheet 6
EZFET_TDO: TP103.1 ; also sheet 6
EZFET_TEST: TP102.1 ; also sheet 6
EZFET_TMS: TP105.1 ; also sheet 6
EZFET_VBUS: C108.1 IC101.1(IN) IC101.6(EN) IC102.6(VCC) J102.1 ; also sheet 5,6
EZFET_VCC: C105.1 IC101.3(OUT) ; also sheet 5,6
GND: C105.2 C108.2 C110.2 C111.2 IC101.2(GND) IC102.3(GND) J102.5 R106.2 R123.2 TP101.1 ; also sheet 5,6
Unconnected: IC102.2(IO2) J102.4

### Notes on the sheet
- USB interface and power supply
- Change IC101 to adjust target voltage from 2.8V to 3.6V
- TLV70033:3.3V
- TLV70033DSE
- DEBUG
- Texas Instruments

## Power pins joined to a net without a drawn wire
P2.3/TA0.0/UCA1STE/A6/C10: MSP1.63(P2.3/TA0.0/UCA1STE/A6/C10)
P2.4/TA1.0/UCA1CLK/A7/C11: MSP1.64(P2.4/TA1.0/UCA1CLK/A7/C11)
P2.7: MSP1.62(P2.7)
P4.5: MSP1.58(P4.5)
P4.6: MSP1.59(P4.6)
P5.4/UCA2TXD/UCA2SIMO/TB0OUTH: MSP1.65(P5.4/UCA2TXD/UCA2SIMO/TB0OUTH)
P6.4/UCB3SIMO/UCB3SDA: MSP1.69(P6.4/UCB3SIMO/UCB3SDA)
P6.5/UCB3SOMI/UCB3SCL: MSP1.70(P6.5/UCB3SOMI/UCB3SCL)
P6.6/UCB3CLK: MSP1.71(P6.6/UCB3CLK)
P6.7/UCB3STE: MSP1.72(P6.7/UCB3STE)
P7.4/TA4.0/A16: MSP1.27(P7.4/TA4.0/A16)
P7.5/A17: MSP1.28(P7.5/A17)
P7.6/A18: MSP1.29(P7.6/A18)
P7.7/A19: MSP1.30(P7.7/A19)
PJ.0/TDO/TB0OUTH/SMCLK/SRSCG1/C6: MSP1.21(PJ.0/TDO/TB0OUTH/SMCLK/SRSCG1/C6)
PJ.1/TDI/TCLK/MCLK/SRSCG0/C7: MSP1.22(PJ.1/TDI/TCLK/MCLK/SRSCG0/C7)
PJ.2/TMS/ACLK/SROSCOFF/C8: MSP1.23(PJ.2/TMS/ACLK/SROSCOFF/C8)
PJ.3/TCK/SRCPUOFF/C9: MSP1.24(PJ.3/TCK/SRCPUOFF/C9)

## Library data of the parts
C1 = MSP430_CapResistor:PANASONIC_SUPERCAP
C2-C9 C12 C13 C101-C103 C105 C107 C108 C110-C125 = rcl:C-EU: CAPACITOR, European symbol
C10 C11 C104 C106 C109 = rcl:CPOL-EU: POLARIZED CAPACITOR, European symbol
D101 D102 = MSP430G6_LP:BAS40-05W
IC101 = roy:TLV70033DSE: 200-mA, Low-I Q , Low-Dropout Regulator for Portable Devices
IC102 = eZFET:TPD4E004
IC103 = roy:TS5A21366RSER: 0.75-Ω DUAL SPST ANALOG SWITCH WITH 1.8-V COMPATIBLE INPUT LOGIC
J1 = LaunchPad_Template_Library:BP_HEADERS_J1
J2 = LaunchPad_Template_Library:BP_HEADERS_J2
J3 = LaunchPad_Template_Library:BP_HEADERS_J3
J4 = LaunchPad_Template_Library:BP_HEADERS_J4
J5 = LaunchPad_Template_Library:BP_HEADERS_PWR_3V3; CCO: 258-0001299; DESCRIPTION: CONN HEADER .100 SINGL STR 3POS; MAN: SULLINS
J6 = LaunchPad_Template_Library:BP_HEADERS_PWR_5V
J7 = MSP430_Headers:JUMPER1X02
J8 = MSP430_Headers:JUMPER1X03
J101 = LaunchPad_Template_Library:J101_2X7_HEADER
J102 = MSP-EXP430G6021:EZFET_MINI-USB-: MINI USB Connector Source: http://www.hirose.co.jp/cataloge_hp/e24000019.pdf
L101 = rcl:L-EU: INDUCTOR, European symbol
LED1 LED2 LED101 LED102 = launchpad:CHIP-LED
MSP1 = MSP_IC:MSP430FR5994
MSP101 = TI_MSP430_v16:F55[0/1/2]X---RGC64: ***F55[0/1/2]X***RGC64 Rev. 1.0 06/2010 "http://www.ti.com/lit/gpn/msp430f5529" "http://www.ti.com/lit/gpn/msp430f5509" F5513/F5514 with limited Functions on some Pins
MSP102 = TI_MSP430_v16:G2X[1/5]2---RSA16: MSP430G2X[1/5]2 MSP430G2x52, MSP430G2x12 QFN (RSA) 16 Pin Package http://focus.ti.com/docs/prod/folders/print/msp430g2452.html
Q1 = MSP_IC:LF_CRYSTAL
Q2 = MSP_Crystals:CRYSTAL
Q101 = MSP430G6_LP:CSTCR4M
R1 = rcl:R-EU_: RESISTOR, European symbol
R2-R5 R7 R101-R109 R112-R128 = resistor:R-US_: RESISTOR, American symbol
R6 = rcl:R-US_: RESISTOR, American symbol
S1-S3 = electricalmeter:PB: OMRON SWITCH
SD1 = Project7264:SD-502702-003: SD-Micro Card connector, Hersteller Molex, H=1,53mm
T101 = MSP430G6_LP:DMG1013UW
T102 = MSP430G6_LP:BC850CW-115
TP101-TP109 = pinhead:PINHD-1X1: PIN HEADER
U$1 = MSP430_Silkscreen:FR5994_REARSILK_REV1_0
U$2 U$3 U$5 U$6 = MSP-EXP432:MOUNTHOLE_125MIL
U$7 = Mike:MIKE_TM
U$8 = LaunchPad_Template_Library:BP_3PIN_SILK
U$10 = LaunchPad_Template_Library:BP_3PIN_SILK_RT

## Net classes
0 default: width 0.254 mm
1 Ground: width 0.305 mm, drill 0.305 mm, clearance 0.152 mm to class 0, clearance 0.152 mm
2 Power: width 0.406 mm, drill 0.305 mm, clearance 0.152 mm to class 0, clearance 0.152 mm to class 1, clearance 0.152 mm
